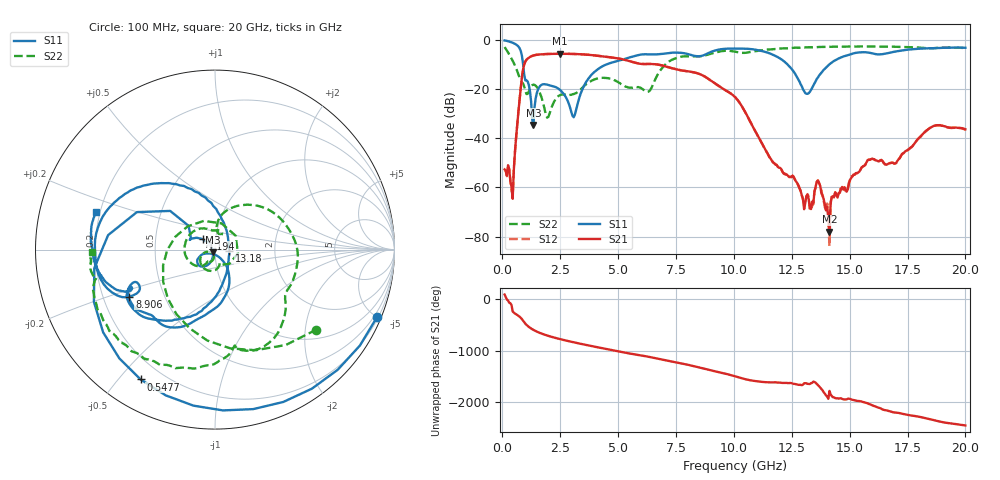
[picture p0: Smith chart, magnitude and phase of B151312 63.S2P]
!  2-Port S-parameters saved by WinCal
! VAR MeasName=S-Parameters (CALIBRATED_DATA) read from VNA (N5244A)
! VAR MeasDate=12/8/2015 5:48:43 PM
! VAR NAME=B151312 63
! VAR FILENAME=B151312 63.S2P
! VAR DATE=12/8/2015 5:48:43 PM
! VAR PHYS_PORTS=1,2
# Hz S DB R 50
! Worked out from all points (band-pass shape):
!   401 points, 100 MHz to 20 GHz, reference 50 ohm
!   highest |S21| = -5.62 dB at 2.488 GHz (marker M1); lowest = -78.0 dB at 14.13 GHz (marker M2)
!   |S21| within 3 dB of the highest: 1.005 GHz to 5.502 GHz (4.497 GHz wide, 138 % of centre)
!   lowest |S11| = -34.5 dB at 1.344 GHz (marker M3), VSWR 1.04, Z = 48.9 - j1.52 ohm
!   |S11| at or under -10 dB: 900.1 MHz to 4.482 GHz (3.582 GHz wide, 133 % of centre); 12.32 GHz to 14.11 GHz (1.792 GHz wide, 13.6 % of centre)
!   |S22| runs from -31.6 to -2.6 dB; largest |S21 - S12| = 0.0017
!   S11 on the Smith chart (normalised r, x): 100 MHz: 0.29, -4.99; 547.8 MHz: 0.12, -0.57; 1.194 GHz: 0.87, +0.10; 8.906 GHz: 0.31, -0.23; 13.18 GHz: 1.17, -0.02; 20 GHz: 0.18, +0.15
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1e8  -0.19 -22.6  -52.65 86.5  -53.15 87.1  -2.85 -38.3
3.985e8  -0.94 -87.2  -59.75 -116.6  -61.09 -114.6  -7.56 -120.9
5.4775e8  -1.58 -119.8  -45.48 78.4  -45.40 78.1  -10.38 -163.0
8.4625e8  -6.33 154.3  -15.39 -29.3  -15.40 -29.4  -17.16 34.0
1.1945e9  -20.85 139.5  -6.92 164.5  -6.92 164.5  -19.73 -80.6
1.34375e9  -34.54 -124.1  -6.30 122.7  -6.30 122.7  -18.18 -109.2
1.94075e9  -18.18 -142.2  -5.71 12.7  -5.71 12.7  -31.60 -133.4
2.488e9  -20.30 -154.9  -5.62 -55.7  -5.62 -55.7  -22.49 -113.3
3.085e9  -31.43 -102.3  -5.68 -118.1  -5.69 -118.1  -21.99 -122.9
3.43325e9  -20.64 -54.5  -5.83 -151.8  -5.83 -151.8  -19.62 -125.4
4.72675e9  -9.21 -94.5  -7.13 92.1  -7.10 92.1  -15.92 144.3
6.7665e9  -5.78 -135.3  -10.08 -79.8  -10.07 -79.9  -13.21 75.2
8.90575e9  -5.30 -151.2  -15.87 68.7  -15.83 68.5  -5.89 -39.1
1.005e10  -3.50 -177.5  -23.21 -56.7  -23.19 -57.0  -4.76 -75.4
1.179125e10  -6.46 128.8  -50.65 -173.0  -50.61 -174.4  -3.66 -96.5
1.318425e10  -21.91 -5.2  -62.99 157.0  -62.67 163.2  -2.95 -115.3
1.338325e10  -19.42 -47.1  -65.73 176.0  -67.47 171.4  -2.99 -117.6
1.3632e10  -15.23 -72.5  -57.25 137.6  -57.03 137.3  -2.90 -121.4
1.41295e10  -9.88 -98.7  -77.95 21.1  -83.87 -23.1  -2.83 -127.0
1.5821e10  -5.12 -152.6  -48.65 130.0  -48.82 128.9  -2.65 -144.7
1.67165e10  -5.24 -154.7  -50.20 -11.4  -50.10 -11.3  -2.69 -152.9
2e10  -3.17 162.5  -36.31 72.1  -36.46 71.6  -3.25 -178.7
